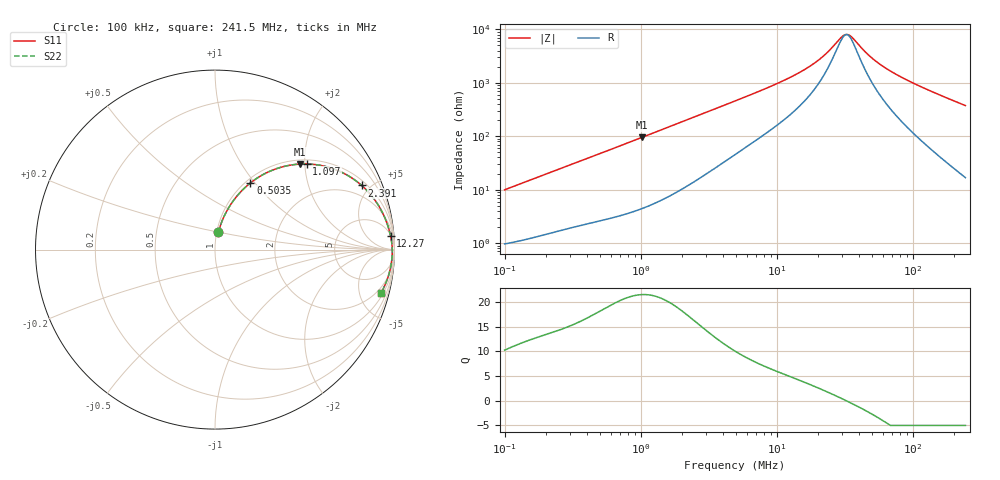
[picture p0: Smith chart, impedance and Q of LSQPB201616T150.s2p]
! LSQPB201616T150  S-PARAMETER MODEL  ( General Type )
! Model Generated by TAIYO YUDEN Corporation (http://www.ty-top.com)
! Version 2.0
! TAIYO YUDEN Control No. 100810NC14SB-FKC
! Copyright(c) 2008 TAIYO YUDEN CO.,LTD. All Rights Reserved.
! Product Description (link to TY-COMPAS)
! https://ds.yuden.co.jp/TYCOMPAS/or/detail?pn=LSQPB201616T150K&u=M
! Products Name : Inductors
! Characteristics :
!  Inductance : 15 uH , SRF(min) : 28 MHz , DC Resistance(max) : 0.78 Ohm
!  Rated Current : Saturation :400 mA , Temp Rise : 410 mA (40 degC)
!  Case Size : 2.0 x 1.6 / 0.079 x 0.063 [mm/inch] , Thickness : 1.6 / 0.063 [mm/inch]
!  (Conditions: Temperature = 25 degC , DC Bias Current/Voltage = 0A / 0V)
! External Node Assignments :
!  1  o---GGG---o  2
! GND o---------o GND
! Frequency Range : 0.1MHz  -  241.513628MHz  [ 402 STEP ]
# MHz S RI R 50
! Freq[MHz].  S11 Real  S11 Imag  S21 Real  S21 Imag  S12 Real  S12 Imag  S22 Real  S22 Imag
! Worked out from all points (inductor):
!   401 points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, 100 kHz to 241.5 MHz, reference 50 ohm
!   read as one part in series: L = 15.7 uH near 104 kHz
!   highest Q = 21.5 at 1.015 MHz (marker M1), where L = 14.8 uH
!   self-resonance near 32.31 MHz
!   S11 on the Smith chart (normalised r, x): 100 kHz: 1.02, +0.20; 503.5 kHz: 1.05, +0.95; 1.097 MHz: 1.10, +2.04; 2.391 MHz: 1.27, +4.43; 12.27 MHz: 6, +24; 241.5 MHz: 1.34, -7.48
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0.1  0.019 0.0961  0.981 -0.0961  0.981 -0.0961  0.019 0.0961
0.213716  0.0543 0.193  0.9457 -0.193  0.9457 -0.193  0.0543 0.193
0.368674  0.1244 0.3006  0.8756 -0.3006  0.8756 -0.3006  0.1244 0.3006
0.503455  0.1973 0.3714  0.8027 -0.3714  0.8027 -0.3714  0.1973 0.3714
0.743203  0.3342 0.448  0.6658 -0.448  0.6658 -0.448  0.3342 0.448
1.014904  0.4742 0.4766  0.5258 -0.4766  0.5258 -0.4766  0.4742 0.4766
1.097121  0.5111 0.4772  0.4889 -0.4772  0.4889 -0.4772  0.5111 0.4772
1.359207  0.6107 0.4643  0.3893 -0.4643  0.3893 -0.4643  0.6107 0.4643
2.39083  0.8171 0.3575  0.1829 -0.3575  0.1829 -0.3575  0.8171 0.3575
3.329076  0.8882 0.2799  0.1118 -0.2799  0.1118 -0.2799  0.8882 0.2799
4.914404  0.9362 0.1997  0.0638 -0.1997  0.0638 -0.1997  0.9362 0.1997
12.27345  0.9784 0.0764  0.0216 -0.0764  0.0216 -0.0764  0.9784 0.0764
18.11814  0.9843 0.0424  0.0157 -0.0424  0.0157 -0.0424  0.9843 0.0424
22.88768  0.9863 0.0246  0.0137 -0.0246  0.0137 -0.0246  0.9863 0.0246
30.06109  0.9875 0.00509  0.0125 -0.00509  0.0125 -0.00509  0.9875 0.00509
32.49632  0.9877 -0.000395  0.0123 0.000395  0.0123 0.000395  0.9877 -0.000395
35.81962  0.9878 -0.00728  0.0122 0.00728  0.0122 0.00728  0.9878 -0.00728
43.52056  0.9876 -0.0213  0.0124 0.0213  0.0124 0.0213  0.9876 -0.0213
49.8765  0.9872 -0.0317  0.0128 0.0317  0.0128 0.0317  0.9872 -0.0317
66.79689  0.9852 -0.0559  0.0148 0.0559  0.0148 0.0559  0.9852 -0.0559
115.2291  0.9749 -0.115  0.0251 0.115  0.0251 0.115  0.9749 -0.115
241.5136  0.924 -0.2435  0.076 0.2435  0.076 0.2435  0.924 -0.2435
